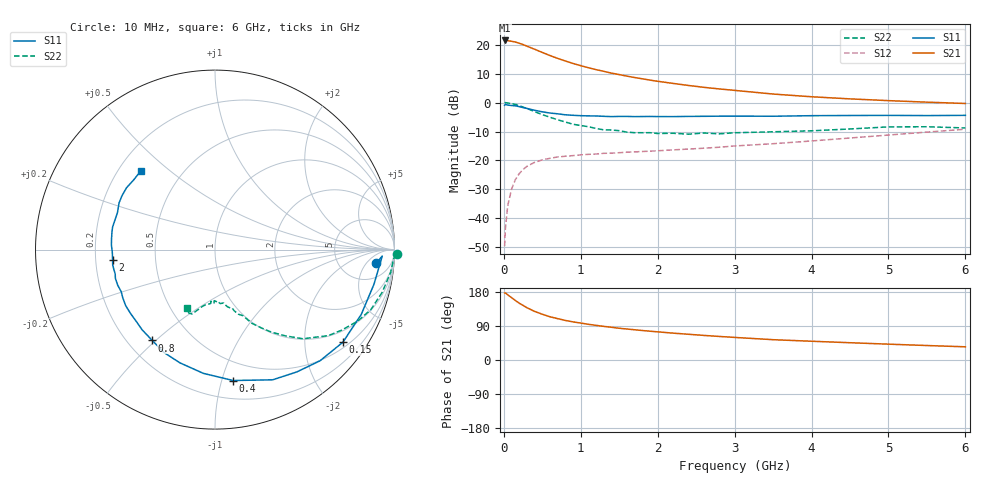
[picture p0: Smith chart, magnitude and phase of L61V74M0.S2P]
!  INFINEON TECHNOLOGIES Small Signal Semiconductors
! BFR380L3 , Si-NPN RF-Transistor in TSLP-3-1
!  Vce=1.75 V,  Ic=4 mA
! Common Emitter S-Parameters:  07. March 2005
#  GHz  S  MA  R  50
! f  S11  S21  S12  S22
! GHz  Mag  Ang  Mag  Ang  Mag  Ang  Mag  Ang
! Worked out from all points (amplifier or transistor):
!   36 points, 10 MHz to 6 GHz, reference 50 ohm
!   highest |S21| = 21.5 dB at 10 MHz (marker M1)
!   |S21| within 3 dB of that: start of sweep to 396.5 MHz
!   unconditionally stable (mu >= 1): 2.502 GHz to 4.756 GHz
!   at 250 MHz: K = 0.14, MSG = 21.6 dB, |S12| = -23.1 dB
!   at 1.4 GHz: K = 0.71, MSG = 13.8 dB, |S12| = -17.5 dB
!   at 6 GHz: K = 0.94, MSG = 4.5 dB, |S12| = -9.2 dB
!   S11 on the Smith chart (normalised r, x): 10 MHz: 12, -9; 150 MHz: 0.65, -2.96; 400 MHz: 0.34, -1.09; 800 MHz: 0.30, -0.49; 2 GHz: 0.27, -0.05; 6 GHz: 0.29, +0.40
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0.01  0.9007 -4.8  11.87 176.8  0.0033 82.0  1.012 -1.5
0.02  0.9326 -2.2  11.82 177.1  0.0066 87.8  0.9962 -3.0
0.05  0.9065 -12.3  11.77 172.1  0.0164 84.4  0.9872 -7.3
0.1  0.8913 -23.9  11.49 164.6  0.0319 78.4  0.9619 -14.2
0.15  0.8798 -35.9  11.13 157.0  0.0467 71.6  0.9305 -21.1
0.2  0.8523 -46.6  10.63 150.0  0.0592 66.5  0.8884 -26.7
0.25  0.82 -56.2  10.06 144.0  0.0699 61.3  0.8368 -32.4
0.3  0.7935 -66.1  9.461 138.0  0.0791 57.3  0.7928 -37.2
0.4  0.7364 -82.1  8.365 128.3  0.0928 50.6  0.6977 -45.4
0.5  0.6925 -95.4  7.363 120.7  0.1023 46.1  0.62 -50.8
0.6  0.6605 -107.2  6.502 114.1  0.109 42.7  0.5575 -55.6
0.8  0.6152 -124.6  5.241 104.4  0.1183 38.9  0.4616 -63.2
0.9  0.6037 -132.3  4.747 100.6  0.1213 37.8  0.4223 -65.6
1.1  0.5899 -143.0  4.009 94.1  0.1276 37.4  0.3828 -70.1
1.5  0.5772 -159.9  3.049 83.8  0.1362 38.3  0.3271 -77.6
2  0.5734 -174.2  2.337 74.3  0.1471 41.4  0.2924 -86.2
2.2  0.5724 -178.5  2.147 70.9  0.1524 43.2  0.2953 -86.5
2.8  0.5828 169.8  1.724 62.2  0.1694 48.6  0.2886 -94.5
3.5  0.5812 159.2  1.406 53.6  0.1948 52.7  0.3131 -100.0
4.5  0.5987 150.1  1.16 45.6  0.2444 58.2  0.3502 -106.1
5.5  0.5967 139.5  1.018 38.2  0.3092 59.6  0.3826 -112.2
6  0.6024 133.3  0.966 34.8  0.3466 58.8  0.3644 -115.8
